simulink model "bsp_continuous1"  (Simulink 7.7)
settings: Solver=ode45  StartTime=0.0  StopTime=25  FixedStep=0.01  RelTol=1e-3
libraries: simulink x1

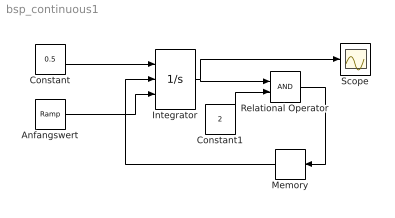
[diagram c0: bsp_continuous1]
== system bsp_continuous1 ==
  Anfangswert : simulink/Sources/Ramp  SystemSampleTime=-1  slope=0.1  start=0  X0=0
  Constant : Constant  Value=0.5
  Constant1 : Constant  Value=2
  Integrator : Integrator  ExternalReset=rising  InitialConditionSource=external  LimitOutput=on  UpperSaturationLimit=2
  Memory : Memory
  Relational Operator : RelationalOperator
  Scope : Scope
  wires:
  Constant/1 -> Integrator/1
  Constant1/1 -> Relational Operator/2
  Integrator/1 -> Relational Operator/1, Scope/1
  Anfangswert/1 -> Integrator/3
  Relational Operator/1 -> Memory/1
  Memory/1 -> Integrator/2
